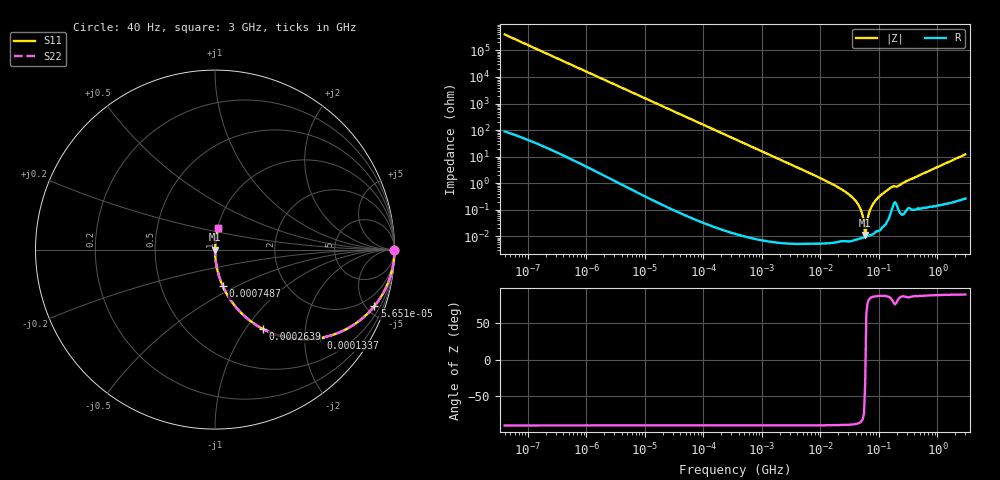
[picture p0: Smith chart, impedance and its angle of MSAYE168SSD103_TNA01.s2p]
! MSAYE168SSD103_TNA01  S-PARAMETER MODEL  ( General Type )
! Model Generated by TAIYO YUDEN Corporation (http://www.ty-top.com)
! Version 2.0
! TAIYO YUDEN Control No. 030711
! Copyright(c) 2003 TAIYO YUDEN CO.,LTD. All Rights Reserved.
! Product Description (link to TY-COMPAS)
! https://ds.yuden.co.jp/TYCOMPAS/or/detail?pn=MSAYE168SSD103KTNA01&u=M
! Products Name : Multilayer Ceramic Capacitors
! Characteristics :
!  Capacitance : 0.01 uF , Rated Voltage : 16V
!  Case Size : 1.6 x 0.8 / 0.063 x 0.031 [mm/inch] , Thickness : 0.8 / 0.031 [mm/inch]
!  (Conditions: Temperature = 25 degC , DC Bias Current/Voltage = 0A / 0V)
! External Node Assignments :
!  1  o---| |---o  2
! GND o---------o GND
! Frequency Range : 40Hz  -  3GHz  [ 401 STEP ]
# MHz S RI R 50
! Freq[MHz].  S11 Real  S11 Imag  S21 Real  S21 Imag  S12 Real  S12 Imag  S22 Real  S22 Imag
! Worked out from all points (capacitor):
!   401 points, 40 Hz to 3 GHz, reference 50 ohm
!   read as one part in series: C = 9.97 nF near 44 Hz
!   lowest |Z| = 11.3 mohm at 58.12 MHz (marker M1)
!   series resonance near 58.77 MHz, so ESL is about 740 pH
!   S11 on the Smith chart (normalised r, x): 40 Hz: open; 56.51 kHz: 1.00, -5.65; 133.7 kHz: 1.00, -2.39; 263.9 kHz: 1.00, -1.21; 748.7 kHz: 1.00, -0.43; 3 GHz: 1.01, +0.24
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4e-05  1 -0.000251  1.19e-07 0.000251  1.19e-07 0.000251  1 -0.000251
0.000834  1 -0.00523  2.87e-05 0.00523  2.87e-05 0.00523  1 -0.00523
0.017386  0.9883 -0.1077  0.0117 0.1077  0.0117 0.1077  0.9883 -0.1077
0.056505  0.8886 -0.3146  0.1114 0.3146  0.1114 0.3146  0.8886 -0.3146
0.133706  0.5875 -0.4922  0.4125 0.4922  0.4125 0.4922  0.5875 -0.4922
0.263915  0.2678 -0.4427  0.7322 0.4427  0.7322 0.4427  0.2678 -0.4427
0.362475  0.1624 -0.3687  0.8376 0.3687  0.8376 0.3687  0.1624 -0.3687
0.748653  0.0435 -0.2038  0.9565 0.2038  0.9565 0.2038  0.0435 -0.2038
1.939641  0.00677 -0.0816  0.9932 0.0816  0.9932 0.0816  0.00677 -0.0816
7.222098  0.000527 -0.0218  0.9995 0.0218  0.9995 0.0218  0.000527 -0.0218
20.48705  0.00011 -0.00685  0.9999 0.00685  0.9999 0.00685  0.00011 -0.00685
35.29647  7.65e-05 -0.00289  0.9999 0.00289  0.9999 0.00289  7.65e-05 -0.00289
46.32945  8.34e-05 -0.0013  0.9999 0.0013  0.9999 0.0013  8.34e-05 -0.0013
50.72622  8.69e-05 -0.000803  0.9999 0.000803  0.9999 0.000803  8.69e-05 -0.000803
55.54024  9.18e-05 -0.000306  0.9999 0.000306  0.9999 0.000306  9.18e-05 -0.000306
58.11596  9.5e-05 -6.06e-05  0.9999 6.06e-05  0.9999 6.06e-05  9.5e-05 -6.06e-05
63.63129  0.000102 0.000424  0.9999 -0.000424  0.9999 -0.000424  0.000102 0.000424
69.67004  0.00011 0.000928  0.9999 -0.000928  0.9999 -0.000928  0.00011 0.000928
83.52119  0.000136 0.00197  0.9999 -0.00197  0.9999 -0.00197  0.000136 0.00197
104.7695  0.000183 0.00338  0.9998 -0.00338  0.9998 -0.00338  0.000183 0.00338
150.5692  0.000571 0.00624  0.9994 -0.00624  0.9994 -0.00624  0.000571 0.00624
3000  0.0171 0.1191  0.9829 -0.1191  0.9829 -0.1191  0.0171 0.1191
